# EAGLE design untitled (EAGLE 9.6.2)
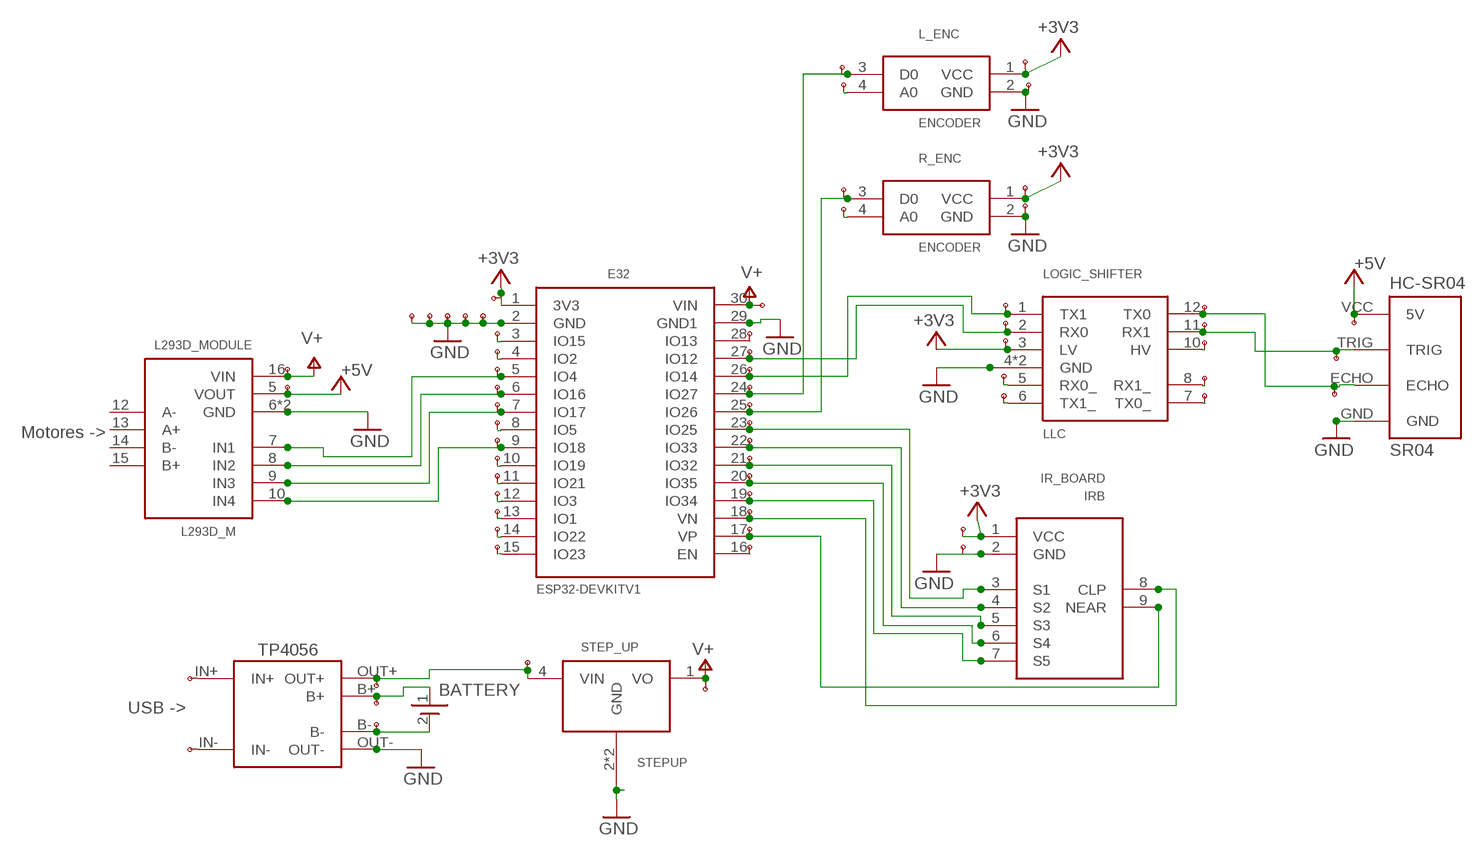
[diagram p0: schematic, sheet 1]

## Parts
BAT_CHARGER  TP4056-MODULE  [TP4056-LITHIUM-PROTECTED-MODULE]
BATTERY  BAT_PAD  [BAT_PAD]
E32  ESP32DEVKITV1  [ESP32-DEVKITV1]
IR_BOARD  IRB  [IRB]
L293D_MODULE  L293D_M  [L293D_M]
L_ENC  ENCODER  [ENCODER]
LOGIC_SHIFTER  LLC  [LLC]
R_ENC  ENCODER  [ENCODER]
SR04  HC-SR04  [HC-SR04_FOOTPRINT]
STEP_UP  STEPUP  [STEPUP]
U$1  TP  [TP]
U$2  TP  [TP]
U$3  TP  [TP]
U$4  TP  [TP]
U$5  TP  [TP]
U$6  TP  [TP]
U$7  TP  [TP]
U$8  TP  [TP]
U$9  TP  [TP]
U$10  TP  [TP]
U$11  TP  [TP]
U$12  TP  [TP]
U$13  TP  [TP]
U$14  TP  [TP]
U$15  TP  [TP]
U$16  TP  [TP]
U$17  TP  [TP]
U$18  TP  [TP]
U$19  TP  [TP]
U$20  TP  [TP]
U$21  TP  [TP]
U$22  TP  [TP]
U$23  TP  [TP]
U$24  TP  [TP]
U$25  TP  [TP]
U$26  TP  [TP]
U$27  TP  [TP]
U$28  TP  [TP]
U$29  TP  [TP]
U$30  TP  [TP]
U$31  TP  [TP]
U$32  TP  [TP]
U$33  TP  [TP]
U$34  TP  [TP]
U$35  TP  [TP]
U$36  TP  [TP]
U$37  TP  [TP]
U$38  TP  [TP]
U$40  TP  [TP]
U$41  TP  [TP]
U$42  TP  [TP]
U$43  TP  [TP]
U$44  TP  [TP]
U$46  TP  [TP]
U$47  TP  [TP]
U$48  TP  [TP]
U$49  TP  [TP]
U$50  TP  [TP]
U$51  TP  [TP]
U$52  TP  [TP]
U$53  TP  [TP]
U$54  TP  [TP]
U$55  TP  [TP]
U$56  TP  [TP]
U$57  TP  [TP]
U$59  TP  [TP]
U$60  TP  [TP]
U$61  TP  [TP]
U$62  TP  [TP]
U$63  TP  [TP]
U$64  TP  [TP]
U$65  TP  [TP]
U$67  TP  [TP]
U$68  TP  [TP]
U$69  TP  [TP]

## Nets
+3V3: E32.1(3V3) IR_BOARD.1(VCC) L_ENC.1(VCC) LOGIC_SHIFTER.3(LV) R_ENC.1(VCC) U$3.P$1 U$8.P$1 U$49.P$1 U$51.P$1 U$57.P$1
+5V: L293D_MODULE.5(VOUT) SR04.VCC(5V) U$2.P$1 U$69.P$1
GND: BAT_CHARGER.OUT- E32.2(GND) E32.29(GND1) IR_BOARD.2(GND) L293D_MODULE.6(GND) L293D_MODULE.11(GND) L_ENC.2(GND) LOGIC_SHIFTER.4(GND) LOGIC_SHIFTER.9(GND) R_ENC.2(GND) SR04.GND STEP_UP.2(GND) STEP_UP.3(GND) U$4.P$1 U$5.P$1 U$6.P$1 U$7.P$1 U$9.P$1 U$35.P$1 U$50.P$1 U$52.P$1
N$1: LOGIC_SHIFTER.12(TX0) SR04.ECHO U$65.P$1 U$67.P$1
N$2: E32.5(IO4) L293D_MODULE.7(IN1) U$46.P$1
N$3: E32.6(IO16) L293D_MODULE.8(IN2) U$12.P$1
N$4: E32.7(IO17) L293D_MODULE.9(IN3) U$13.P$1
N$5: E32.9(IO18) L293D_MODULE.10(IN4) U$15.P$1
N$6: BAT_CHARGER.B+ BATTERY.1(+) U$41.P$1
N$7: BAT_CHARGER.B- BATTERY.2(-) U$40.P$1
N$8: BAT_CHARGER.OUT+ STEP_UP.4(VIN) U$42.P$1 U$43.P$1
N$9: E32.23(IO25) IR_BOARD.3(S1) U$29.P$1
N$10: E32.22(IO33) IR_BOARD.4(S2) U$28.P$1
N$11: E32.21(IO32) IR_BOARD.5(S3) U$27.P$1
N$12: E32.20(IO35) IR_BOARD.6(S4) U$26.P$1
N$13: E32.19(IO34) IR_BOARD.7(S5) U$25.P$1
N$14: E32.17(VP) IR_BOARD.9(NEAR) U$23.P$1
N$15: E32.18(VN) IR_BOARD.8(CLP) U$24.P$1
N$16: E32.27(IO12) LOGIC_SHIFTER.2(RX0) U$33.P$1 U$56.P$1
N$17: E32.26(IO14) LOGIC_SHIFTER.1(TX1) U$32.P$1 U$55.P$1
N$18: LOGIC_SHIFTER.11(RX1) SR04.TRIG U$64.P$1 U$68.P$1
N$21: E32.24(IO27) L_ENC.3(D0) U$31.P$1 U$47.P$1
N$22: E32.15(IO23) U$21.P$1
N$23: E32.3(IO15) U$10.P$1
N$24: E32.4(IO2) U$11.P$1
N$25: E32.8(IO5) U$14.P$1
N$26: E32.10(IO19) U$16.P$1
N$27: E32.11(IO21) U$17.P$1
N$28: E32.12(IO3) U$18.P$1
N$29: E32.13(IO1) U$19.P$1
N$30: E32.14(IO22) U$20.P$1
N$31: E32.25(IO26) R_ENC.3(D0) U$30.P$1 U$54.P$1
N$32: E32.16(EN) U$22.P$1
N$33: E32.28(IO13) U$34.P$1
N$35: BAT_CHARGER.IN- U$38.P$1
N$36: BAT_CHARGER.IN+ U$37.P$1
N$37: LOGIC_SHIFTER.5(RX0_) U$59.P$1
N$38: LOGIC_SHIFTER.6(TX1_) U$60.P$1
N$39: LOGIC_SHIFTER.7(TX0_) U$61.P$1
N$40: LOGIC_SHIFTER.8(RX1_) U$62.P$1
N$41: LOGIC_SHIFTER.10(HV) U$63.P$1
N$42: R_ENC.4(A0) U$53.P$1
N$43: L_ENC.4(A0) U$48.P$1
V+: E32.30(VIN) L293D_MODULE.16(VIN) STEP_UP.1(VO) U$1.P$1 U$36.P$1 U$44.P$1
Unconnected: L293D_MODULE.12(A-) L293D_MODULE.13(A+) L293D_MODULE.14(B-) L293D_MODULE.15(B+)

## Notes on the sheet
- Motores ->
- TP4056
- USB ->

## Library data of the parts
BAT_CHARGER = UserLib:TP4056-MODULE
BATTERY = edurobotParts:BAT_PAD
E32 = ESP32-DEVKITV1:ESP32DEVKITV1
IR_BOARD = edurobotParts:IRB
L293D_MODULE = edurobotParts:L293D_M
L_ENC R_ENC = edurobotParts:ENCODER
LOGIC_SHIFTER = edurobotParts:LLC
SR04 = Ultrasonic Sensor HC-SR04:HC-SR04: Ultrasonic Sensor HC-SR04
STEP_UP = edurobotParts:STEPUP
U$1-U$38 U$40-U$44 U$46-U$57 U$59-U$65 U$67-U$69 = edurobotParts:TP

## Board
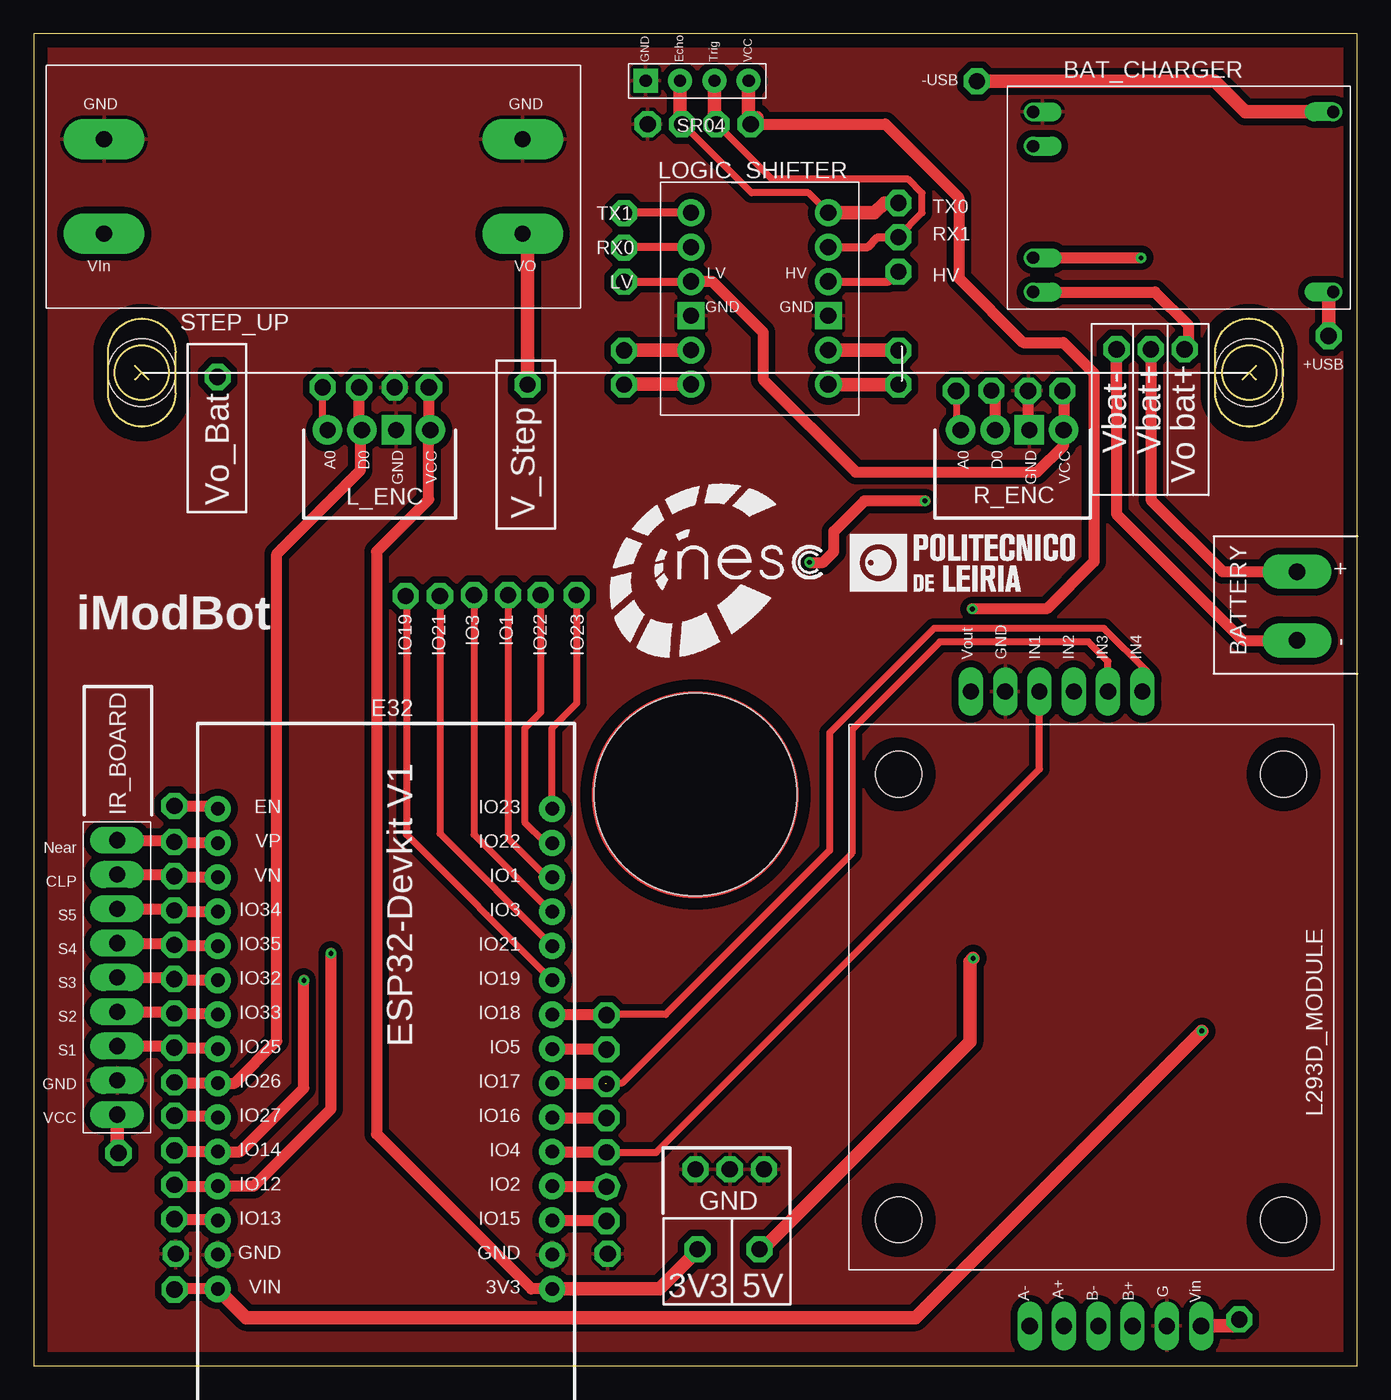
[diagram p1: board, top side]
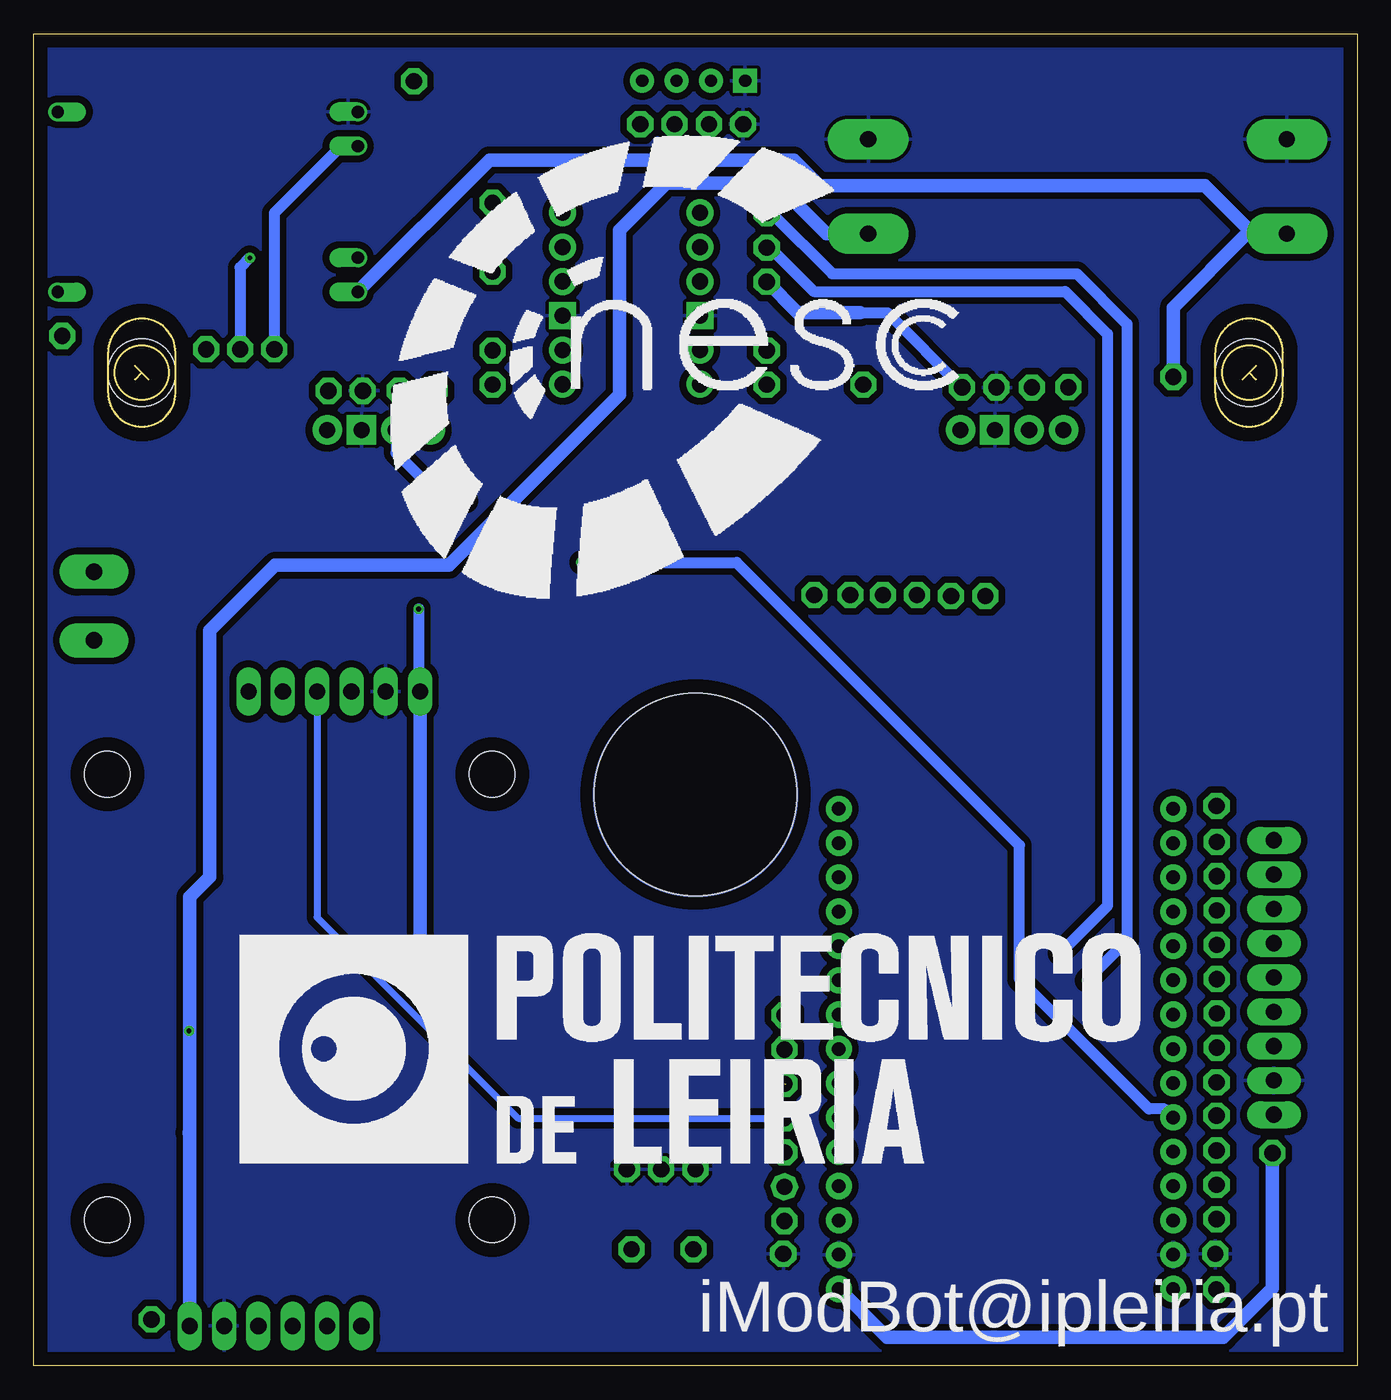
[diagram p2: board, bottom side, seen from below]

Size 98 x 98.64 mm. Coordinates in mm from the lower left corner, seen from the top.
Outline: 7.5,74.04 8,73.54
Outline: 8,73.54 8.5,73.04
Outline: 8,73.54 7.5,73.04
Outline: 90,73.54 90.5,73.04
Outline: 90.5,74.04 90,73.54
Outline: 90,73.54 89.5,73.04
Outline: 0,0 98,0 98,98.64 0,98.64 0,0
Outline: 5.5,72.04 5.5,75.04 arc-180 10.5,75.04 10.5,72.04 arc-180 5.5,72.04
Outline: 87.5,72.04 87.5,75.04 arc-180 92.5,75.04 92.5,72.04 arc-180 87.5,72.04
Outline: circle at 8,73.54 radius 2
Outline: circle at 90,73.54 radius 2
Copper layers (1*16): Top 0.035mm / dielectric 1.5mm / Bottom 0.035mm
Design rules "default *": minimum track width 6mil, minimum drill 0.35mm, track to track 0.5mm, track to pad 0.54mm, pad to pad 0.2mm, via to via 0.2mm, smd to smd 6mil, copper to edge 40mil, drill to drill 6mil, minimum pad ring 10mil, minimum via ring 8mil, stop-mask expansion 0.1mm, vias tented up to drill 0mil, thermal gap 10mil
Holes 15 mm at 49,42.29
Holes 5 mm at 8,73.54 90,73.54

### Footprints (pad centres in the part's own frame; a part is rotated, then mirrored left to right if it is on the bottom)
TP4056-LITHIUM-PROTECTED-MODULE = drill 0.9 offset: B+ 10.795,4.445; B- 10.795,-3.81; IN+ -11.43,6.985; IN- -11.43,-6.35; OUT+ 10.795,6.985; OUT- 10.795,-6.35
BAT_PAD = drill 1.2 pad 2.54 long: 1 0,2.54; 2 0,-2.54
ESP32-DEVKITV1 = drill 1 pad 1.93: 1 -22.87,-13.54; 2 -20.33,-13.54; 3 -17.79,-13.54; 4 -15.25,-13.54; 5 -12.71,-13.54; 6 -10.17,-13.54; 7 -7.63,-13.54; 8 -5.09,-13.54; 9 -2.55,-13.54; 10 -0.01,-13.54; 11 2.53,-13.54; 12 5.07,-13.54; 13 7.61,-13.54; 14 10.15,-13.54; 15 12.69,-13.54; 16 12.69,11.23; 17 10.15,11.23; 18 7.61,11.23; 19 5.07,11.23; 20 2.53,11.23; 21 -0.01,11.23; 22 -2.55,11.23; 23 -5.09,11.23; 24 -7.63,11.23; 25 -10.17,11.23; 26 -12.71,11.23; 27 -15.25,11.23; 28 -17.79,11.23; 29 -20.33,11.23; 30 -22.87,11.23
IRB = drill 1.2 pad 2 long: 1 -10.16,0; 2 -7.62,0; 3 -5.08,0; 4 -2.54,0; 5 0,0; 6 2.54,0; 7 5.08,0; 8 7.62,0; 9 10.16,0
L293D_M = drill 1.2 long: 5 24.13,8.16; 6 24.13,5.62; 7 24.13,3.08; 8 24.13,0.54; 9 24.13,-2; 10 24.13,-4.54; 11 -22.86,-6.35; 12 -22.86,3.81; 13 -22.86,1.27; 14 -22.86,-1.27; 15 -22.86,-3.81; 16 -22.86,-8.89 | hole 3.4: -15,-15; 18,-15; -15,13.5; 18,13.5
ENCODER = drill 1.2 pad 2.184: 1 0,3.81; 3 0,-1.27; 4 0,-3.81 | drill 1.2 pad 2.184 square: 2 0,1.27
LLC = drill 1.2 pad 2: 1 -5.08,5.08; 2 -5.08,2.54; 3 -5.08,0; 5 -5.08,-5.08; 6 -5.08,-7.62; 7 5.08,-7.62; 8 5.08,-5.08; 10 5.08,0; 11 5.08,2.54; 12 5.08,5.08 | drill 1.2 pad 2 square: 4 -5.08,-2.54; 9 5.08,-2.54
HC-SR04_FOOTPRINT = drill 0.9 pad 1.778: ECHO 0,1.27; TRIG 0,-1.27; VCC 0,-3.81 | drill 0.9 pad 1.778 square: GND 0,3.81
STEPUP = drill 1.2 pad 3 long: 1 -15.5,3.5; 2 -15.5,-3.5; 3 15.5,-3.5; 4 15.5,3.5
TP = drill 1.2 pad 1.93 octagon: P$1 0,0

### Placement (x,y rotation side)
BAT_CHARGER  84.8,86.5 180 top
BATTERY  93.54,56.26 0 top
E32  24.85,28.55 90 top
IR_BOARD  6.17,28.75 90 top
L293D_MODULE  77.56,25.8 90 top
L_ENC  25.56,69.29 270 top
LOGIC_SHIFTER  53.75,80.3 0 top
R_ENC  72.45,69.29 270 top
SR04  49.13,95.15 90 top
STEP_UP  20.7,87.32 180 top
U$1  89.28,3.43 0 top
U$2  53.73,8.63 0 top
U$3  76.18,72.19 0 top
U$4  73.64,72.19 0 top
U$5  49,14.54 0 top
U$6  10.5,8.29 0 top
U$7  54.08,14.54 0 top
U$8  43.72,80.26 0 top
U$9  42.5,8.29 0 top
U$10  42.42,10.72 90 top
U$11  42.42,13.26 70.3 top
U$12  42.42,18.34 0 top
U$13  42.42,20.88 0 top
U$14  42.42,23.42 0 top
U$15  42.42,25.96 90 top
U$16  27.53,57 0 top
U$17  30.07,57 0 top
U$18  32.59,57.08 0 top
U$19  35.13,57.08 0 top
U$20  37.54,57.08 0 top
U$21  40.2,57.07 0 top
U$22  10.41,41.45 0 top
U$23  10.39,38.79 90 top
U$24  10.39,36.25 90 top
U$25  10.39,33.71 90 top
U$26  10.39,31.17 90 top
U$27  10.39,28.63 90 top
U$28  10.39,26.09 90 top
U$29  10.39,23.55 0 top
U$30  70.92,72.21 0 top
U$31  24.1,72.44 0 top
U$32  10.41,15.94 0 top
U$33  10.41,13.4 0 top
U$34  10.41,10.86 0 bottom
U$35  51.54,14.54 0 top
U$36  36.58,72.64 0 top
U$37  95.89,76.26 0 top
U$38  69.85,95.12 0 top
U$40  80.19,75.27 0 top
U$41  82.72,75.27 0 bottom
U$42  85.22,75.27 0 top
U$43  13.61,73.23 0 top
U$44  10.42,5.64 0 top
U$46  42.42,15.8 0 top
U$47  10.41,20.98 0 top
U$48  21.38,72.46 0 top
U$49  49.16,8.63 0 top
U$50  45.47,91.95 0 top
U$51  29.25,72.45 0 top
U$52  26.71,72.45 0 top
U$53  68.31,72.19 0 top
U$54  10.41,18.52 0 top
U$55  43.72,85.34 0 top
U$56  43.72,82.8 0 top
U$57  6.27,15.75 90 top
U$59  43.72,75.18 0 top
U$60  43.72,72.64 0 top
U$61  64.02,72.64 0 top
U$62  64.02,75.18 0 top
U$63  64.02,81.03 0 top
U$64  64.02,83.57 0 top
U$65  64.02,86.11 0 top
U$67  48.01,91.95 0 top
U$68  50.55,91.95 0 top
U$69  53.09,91.95 0 top

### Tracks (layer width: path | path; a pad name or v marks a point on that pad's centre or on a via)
+3V3
  Top 0.61: U$8.P$1 43.75,80.3 LOGIC_SHIFTER.3
  Top 0.813: 76.39,71.98 U$3.P$1 76.27,72.11 R_ENC.1 76.27,68.15 74.28,66.16 60.88,66.16 54,73.04 54,76.54 50.24,80.3 LOGIC_SHIFTER.3 | U$51.P$1 29.25,69.41 | 29.25,69.41 L_ENC.1 | E32.1 36.86,5.68 25.38,17.16 25.38,60.29 29.25,64.16 29.25,69.41
  Top 1.016: U$49.P$1 49.16,8.5 46.34,5.68 E32.1 | IR_BOARD.1 6.17,15.85 U$57.P$1
  Bottom 0.813: 36.82,77.98 34.78,77.98 U$51.P$1
  Bottom 1.016: U$57.P$1 6.27,5.74 9.91,2.1 34.81,2.1 E32.1 | U$8.P$1 41.43,77.98 36.82,77.98
+5V  (via drill 0.35)
  Top 0.813: U$69.P$1 63.05,91.95 68.5,86.5 68.5,80.54 73.26,75.78 76.24,75.78 78.51,73.5 78.51,59.54 75.01,56.04 v69.5,56.04
  Top 1.016: SR04.VCC 52.94,92.09 U$69.P$1 53.56,92.42 | v69.56,30.17 69.31,29.92 69.31,23.97 53.97,8.63 U$2.P$1
  Bottom 0.813: v69.5,56.04 69.5,50.03 L293D_MODULE.5
  Bottom 1.016: L293D_MODULE.5 69.4,30.33 v69.56,30.17
GND
  Top 0.813: R_ENC.2 73.64,69.38 U$4.P$1
  pour Top: 0,0 98,0 98,98.64 0,98.64
  pour Bottom: 0,0 98.04,0 98.04,98.68 0,98.68
N$1
  Top 0.508: LOGIC_SHIFTER.12 57.35,86.86 53.15,86.86 47.91,92.09 47.86,92.09
  Top 1.016: SR04.ECHO 47.86,92.09 U$67.P$1 | LOGIC_SHIFTER.12 62.26,85.38 62.99,86.11 U$65.P$1
N$2
  Top 0.508: U$46.P$1 46.09,15.8 74.48,44.19 L293D_MODULE.7
  Top 0.813: E32.5 42.37,15.84 U$46.P$1
N$3
  Top 0.813: U$12.P$1 38.44,18.34 E32.6
  Bottom 0.508: L293D_MODULE.8 77.02,33.2 62.15,18.34 U$12.P$1
N$4  (1 unrouted)
  Top 0.152: U$13.P$1 42.37,20.92
  Top 0.508: L293D_MODULE.9 79.56,52.15 78.11,53.6 67.09,53.6 60.58,47.09 60.58,37.95 43.55,20.92 42.37,20.92
  Top 0.813: E32.7 42.37,20.92 | 42.29,20.88 42.24,20.92
N$5
  Top 0.508: L293D_MODULE.10 82.1,51.07 82.45,51.42 79.25,54.61 66.67,54.61 58.94,46.87 58.94,38.14 46.8,26 42.37,26
  Top 0.813: E32.9 42.37,26 U$15.P$1
N$6  (via drill 0.35)
  Top 0.813: 82.72,73.55 U$41.P$1 82.72,64.12 88.04,58.8 BATTERY.1 | BAT_CHARGER.B+ 81.99,82.05 v82,82.04
  Bottom 0.813: v82,82.04 82.72,81.32 U$41.P$1
N$7
  Top 0.813: 80.19,72.48 U$40.P$1 80.19,63.07 89.54,53.72 BATTERY.2
  Bottom 0.813: BAT_CHARGER.B- 75.23,90.31 80.19,85.36 U$40.P$1
N$8
  Top 0.813: BAT_CHARGER.OUT+ 83.03,79.51 85.5,77.04 85.5,75.55 U$42.P$1
  Bottom 1.016: U$43.P$1 13.61,78.37 8.15,83.82 STEP_UP.4 7.74,83.82 11.3,87.38 39.81,87.38 41.72,89.28 64.26,89.28 74,79.54 BAT_CHARGER.OUT+
N$9
  Top 0.813: IR_BOARD.3 10.27,23.67 U$29.P$1 13.53,23.55 E32.23
N$10
  Top 0.152: E32.22 10.71,26 10.5,26.21
  Top 0.305: U$28.P$1 11.43,26.09
  Top 0.813: IR_BOARD.4 10.5,26.21 10.92,26.21 | 11.43,26.09 13.53,26.09 E32.22
N$11
  Top 0.813: E32.21 10.48,28.54 U$27.P$1 10.27,28.75 IR_BOARD.5
N$12
  Top 0.813: E32.20 10.48,31.08 U$26.P$1 10.27,31.29 IR_BOARD.6
N$13
  Top 0.813: IR_BOARD.7 10.27,33.83 U$25.P$1 10.48,33.62 E32.19
N$14
  Top 0.813: IR_BOARD.9 10.27,38.91 U$23.P$1 10.48,38.7 E32.17
N$15
  Top 0.813: IR_BOARD.8 10.27,36.37 U$24.P$1 10.48,36.16 E32.18
N$16  (via drill 0.35)
  Top 0.61: LOGIC_SHIFTER.2 43.75,82.84 U$56.P$1
  Top 0.813: U$33.P$1 10.51,13.3 E32.27 16.3,13.3 22,19 v22,30.54
  Bottom 0.813: U$56.P$1 43.5,82.8 40.23,79.54 21.62,79.54 18.48,76.41 18.48,34.05 v22,30.54
N$17  (via drill 0.35)
  Top 0.61: LOGIC_SHIFTER.1 43.75,85.38 U$55.P$1
  Top 0.813: U$32.P$1 10.51,15.84 E32.26 15.29,15.84 20,20.56 v20,28.54
  Bottom 0.813: U$55.P$1 43.36,85.34 38.87,80.85 20.75,80.85 17.05,77.15 17.05,31.49 v20,28.54
N$18
  Top 0.508: 50.4,92.09 50.45,92.09 54.68,87.87 64.75,87.87 65.78,86.84 65.78,85.38 64.02,83.62 U$64.P$1
  Top 0.61: LOGIC_SHIFTER.11 61.75,82.84 62.48,83.57 U$64.P$1
  Top 1.016: SR04.TRIG 50.4,92.09 U$68.P$1
N$21
  Top 0.813: U$47.P$1 10.47,20.92 E32.24 14.88,20.92 18,24.04 18,60.12 24.17,66.29 24.17,69.22 24.6,68.79 24.6,68.98 L_ENC.3 24.1,69.49 U$31.P$1
N$22
  Top 0.508: E32.15 38.39,47.24 40.2,49.05 U$21.P$1
N$23
  Top 0.813: E32.3 42.37,10.76 U$10.P$1
N$24
  Top 0.813: U$11.P$1 38.44,13.26 E32.4
N$25
  Top 0.813: U$14.P$1 38.44,23.42 E32.8
N$26
  Top 0.508: E32.10 27.6,39.34 27.6,56.94 U$16.P$1
  Top 0.813: 27.49,57.05 U$16.P$1
N$27
  Top 0.508: E32.11 30.07,39.4 U$17.P$1
  Top 0.813: 38.44,31.04 E32.11
N$28
  Top 0.508: 38.44,33.58 38.35,33.58 32.59,39.34 U$18.P$1
  Top 0.813: 38.44,33.58 E32.12
N$29
  Top 0.508: E32.13 38,36.16 35.13,39.03 U$19.P$1
  Top 0.813: E32.13 37.76,36.16
N$30
  Top 0.508: E32.14 37.89,38.7 36.36,40.23 36.36,47.2 37.54,48.38 U$20.P$1
N$31  (via drill 0.35)
  Top 0.813: 10.51,18.42 U$54.P$1 13.49,18.52 E32.25 13.67,18.34 | v66,64.04 61.5,64.04 59.25,61.79 59.25,60.29 58.45,59.49 v57.45,59.49 | U$30.P$1 71.19,71.95 R_ENC.3
  Bottom 0.813: R_ENC.3 71.19,67.61 67.62,64.04 v66,64.04 | v57.45,59.49 45.95,59.49 25,38.54 25,28.6 15.41,19.01 14.25,19.01 E32.25
N$32
  Top 0.813: U$22.P$1 13.41,41.45 E32.16
N$33
  Top 0.813: U$34.P$1 13.53,10.86 E32.28
N$35
  Top 1.016: U$38.P$1 87.45,95.12 89.73,92.85 BAT_CHARGER.IN-
N$36
  Top 1.016: U$37.P$1 95.89,79.17 BAT_CHARGER.IN+
N$37
  Top 1.016: U$59.P$1 43.75,75.22 LOGIC_SHIFTER.5
N$38
  Top 1.016: LOGIC_SHIFTER.6 43.75,72.68 U$60.P$1
N$39
  Top 1.016: U$61.P$1 58.87,72.64 LOGIC_SHIFTER.7
N$40
  Top 1.016: LOGIC_SHIFTER.8 63.99,75.22 U$62.P$1
N$41
  Top 0.61: LOGIC_SHIFTER.10 63.29,80.3 U$63.P$1
N$42
  Top 0.508: U$53.P$1 68.31,69.63 R_ENC.4
N$43
  Top 0.508: L_ENC.4 21.38,69.66 U$48.P$1
V+  (via drill 0.35)
  Top 0.152: E32.30 13.41,5.89
  Top 0.813: E32.30 10.46,5.68 U$44.P$1 | 86.5,24.78 v86.5,24.79
  Top 1.016: STEP_UP.1 36.58,83.45 U$36.P$1 | 13.41,5.89 15.74,3.56 65.29,3.56 86.5,24.78 | U$1.P$1 88.79,2.94 L293D_MODULE.16
  Bottom 0.813: 86.45,23.54 86.45,24.74 v86.5,24.79
  Bottom 1.016: STEP_UP.1 39.31,83.82 43.05,87.57 51.14,87.57 54.61,84.09 54.61,71.93 67.25,59.29 80.11,59.29 84.96,54.44 84.96,36.2 86.45,34.71 86.45,23.54 L293D_MODULE.16 86.45,17.11 86.49,17.27
(copper drawn outside any net)
  shapes: Bottom circle x1, Top circle x1

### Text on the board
tPlace: -USB | TX0 | TX1 | RX1 | RX0 | HV | LV | Vbat+ | Vo bat+ | +USB | Vbat- | Vo_Bat | V_Step | IO3 | IO1 | IO19 | IO21 | IO22 | IO23 | GND | 3V3 | 5V
bPlace: iModBot@ipleiria.pt
tNames: iModBot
